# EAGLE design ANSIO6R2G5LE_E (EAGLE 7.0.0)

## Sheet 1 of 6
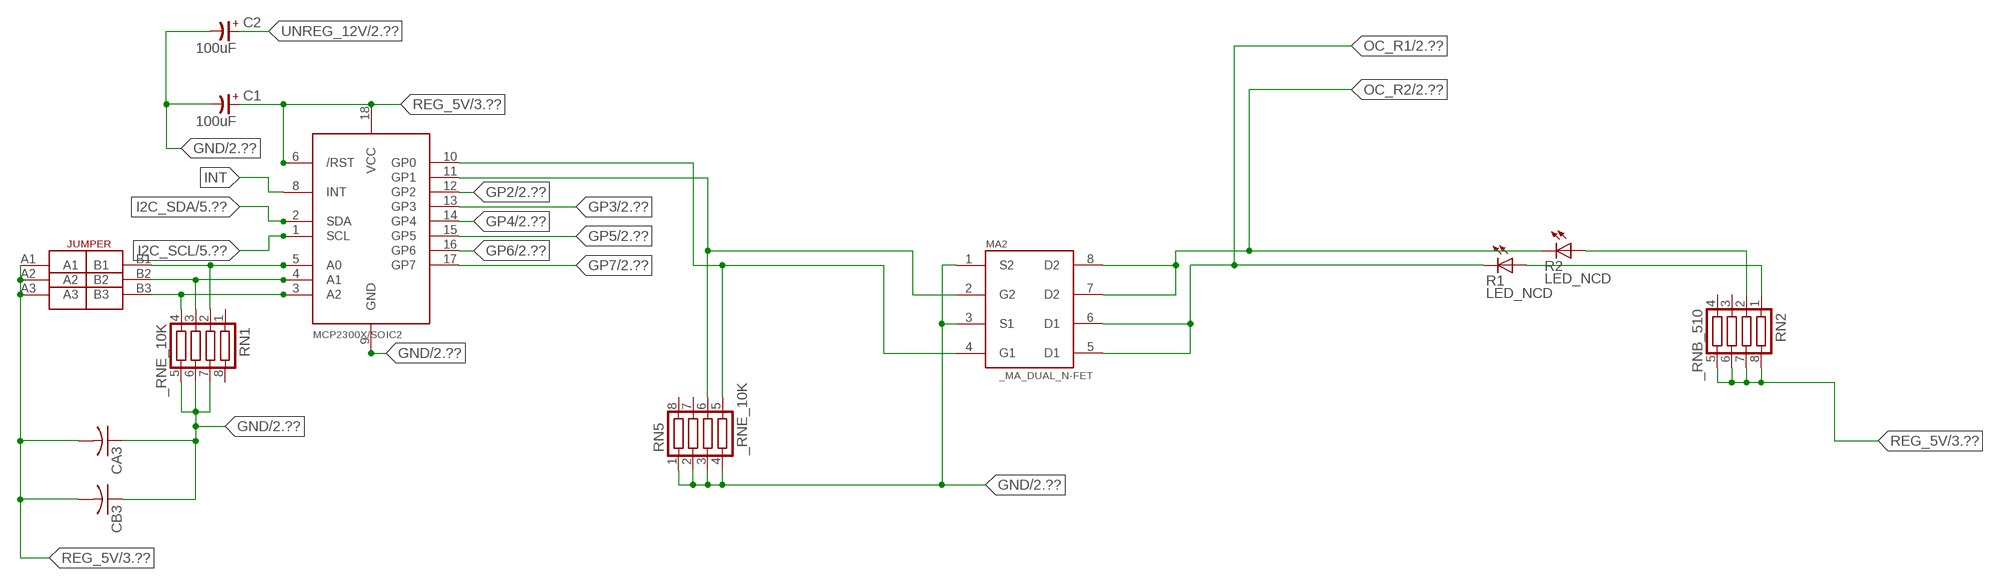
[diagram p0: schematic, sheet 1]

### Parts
C1  100uF  CP-E-025X060  [E-025X060]
C2  100uF  CP-E-025X060  [E-025X060]
CA3  CC1206KRX7R9BB104C1206K  [CC1206KRX7R9BB104]
CB3  TMK316F106ZL-TC1206K  [TMK316F106ZL-T]
IC2  MCP2300X/SO  [SO18W]
MA2  _MA_DUAL_N-FET  [_MA_DUAL_N-FET]
R1  LED_NCD  [CHIPLED_0603]
R2  LED_NCD  [CHIPLED_0603]
RN1  _RNE_10K  [RNE]
RN2  _RNB_510  [RNB]
RN5  _RNE_10K  [RNE]
U$18  JUMPER_3X2  [JUMPER_3X2]

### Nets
GND: C1.- C2.- CA3.1 CB3.1 IC2.9(GND) MA2.1(S2) MA2.3(S1) RN1.5 RN1.6 RN1.7 RN5.1 RN5.2 RN5.3 RN5.4 ; also sheet 2,3,4,5,6
GP2: IC2.12(GP2) ; also sheet 2
GP3: IC2.13(GP3) ; also sheet 2
GP4: IC2.14(GP4) ; also sheet 2
GP5: IC2.15(GP5) ; also sheet 2
GP6: IC2.16(GP6) ; also sheet 2
GP7: IC2.17(GP7) ; also sheet 2
I2C_SCL: IC2.1(SCL) ; also sheet 5,6
I2C_SDA: IC2.2(SDA) ; also sheet 5,6
INT: IC2.8(INT)
N$6: IC2.5(A0) RN1.2 U$18.B1
N$7: IC2.4(A1) RN1.3 U$18.B2
N$8: IC2.3(A2) RN1.4 U$18.B3
N$22: IC2.11(GP1) MA2.2(G2) RN5.6
N$23: IC2.10(GP0) MA2.4(G1) RN5.5
N$31: R2.A RN2.2
N$32: R1.A RN2.1
OC_R1: MA2.5(D1) MA2.6(D1) R1.C ; also sheet 2
OC_R2: MA2.7(D2) MA2.8(D2) R2.C ; also sheet 2
REG_5V: C1.+ CA3.2 CB3.2 IC2.6(/RST) IC2.18(VCC) RN2.5 RN2.6 RN2.7 RN2.8 U$18.A1 U$18.A2 U$18.A3 ; also sheet 3,4,5,6
UNREG_12V: C2.+ ; also sheet 2,3
Unconnected: RN1.1 RN1.8 RN2.3 RN2.4 RN5.7 RN5.8

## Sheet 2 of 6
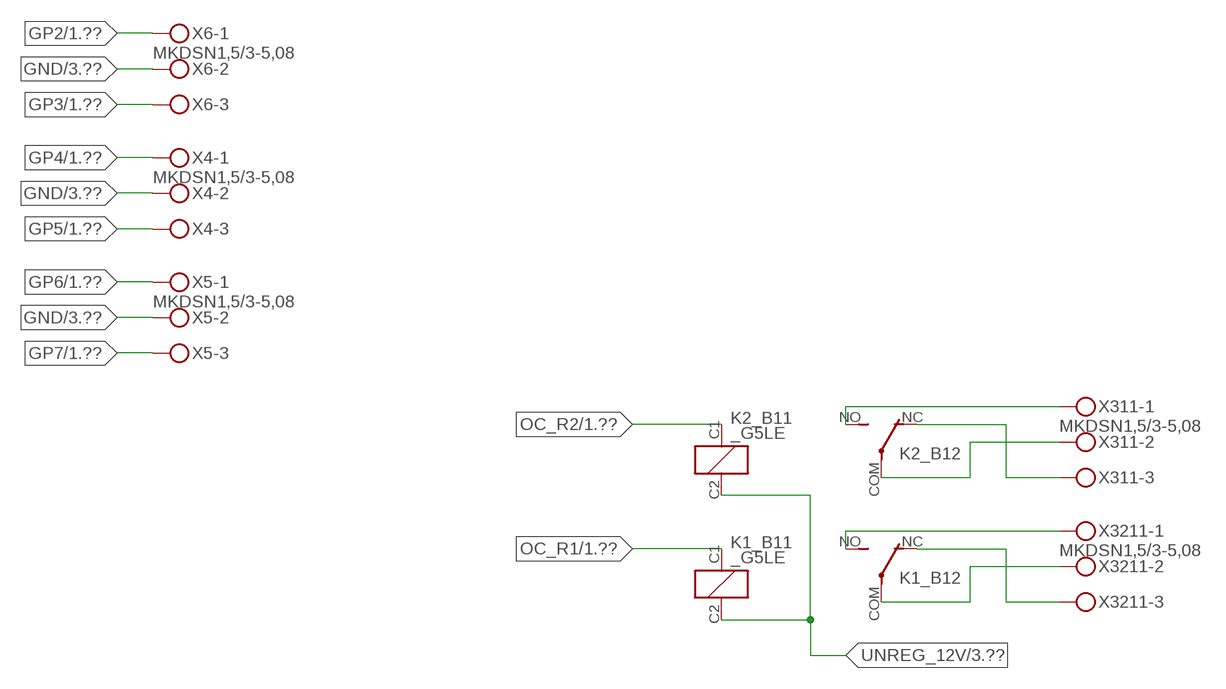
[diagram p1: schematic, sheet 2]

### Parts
K1_B1  _G5LE  [G5LE]
K2_B1  _G5LE  [G5LE]
X4  MKDSN1,5/3-5,08  [MKDSN1,5/3-5,08]
X5  MKDSN1,5/3-5,08  [MKDSN1,5/3-5,08]
X6  MKDSN1,5/3-5,08  [MKDSN1,5/3-5,08]
X311  MKDSN1,5/3-5,08  [MKDSN1,5/3-5,08]
X3211  MKDSN1,5/3-5,08  [MKDSN1,5/3-5,08]

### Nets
GND: X4.2 X5.2 X6.2 ; also sheet 1,3,4,5,6
GP2: X6.1 ; also sheet 1
GP3: X6.3 ; also sheet 1
GP4: X4.1 ; also sheet 1
GP5: X4.3 ; also sheet 1
GP6: X5.1 ; also sheet 1
GP7: X5.3 ; also sheet 1
N$221: K2_B1.NO(2:NO) X311.1
N$222: K2_B1.NC(2:NC) X311.3
N$223: K2_B1.COM(2:COM) X311.2
N$224: K1_B1.NO(2:NO) X3211.1
N$225: K1_B1.NC(2:NC) X3211.3
N$226: K1_B1.COM(2:COM) X3211.2
OC_R1: K1_B1.C1(1:C1) ; also sheet 1
OC_R2: K2_B1.C1(1:C1) ; also sheet 1
UNREG_12V: K1_B1.C2(1:C2) K2_B1.C2(1:C2) ; also sheet 1,3

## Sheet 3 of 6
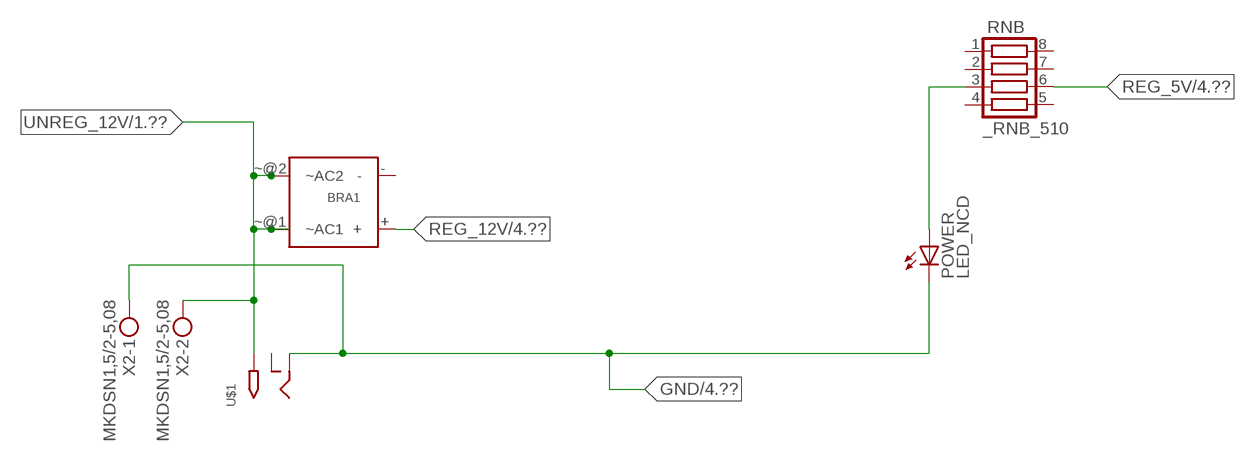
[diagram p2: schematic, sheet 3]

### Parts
BRA1  MB2S_  [MB2S]
POWER  LED_NCD  [CHIPLED_0603]
RNB  _RNB_510  [RNB]
U$1  2.1MMJACK  [PJ-102A]
X2  MKDSN1,5/2-5,08  [MKDSN1,5/2-5,08]

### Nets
GND: POWER.C U$1.RING X2.1 ; also sheet 1,2,4,5,6
N$1: POWER.A RNB.3
REG_5V: RNB.6 ; also sheet 1,4,5,6
REG_12V: BRA1.+ ; also sheet 4
UNREG_12V: BRA1.~@1(~AC1) BRA1.~@2(~AC2) U$1.TIP X2.2 ; also sheet 1,2
Unconnected: BRA1.- RNB.1 RNB.2 RNB.4 RNB.5 RNB.7 RNB.8 U$1.RING_SW

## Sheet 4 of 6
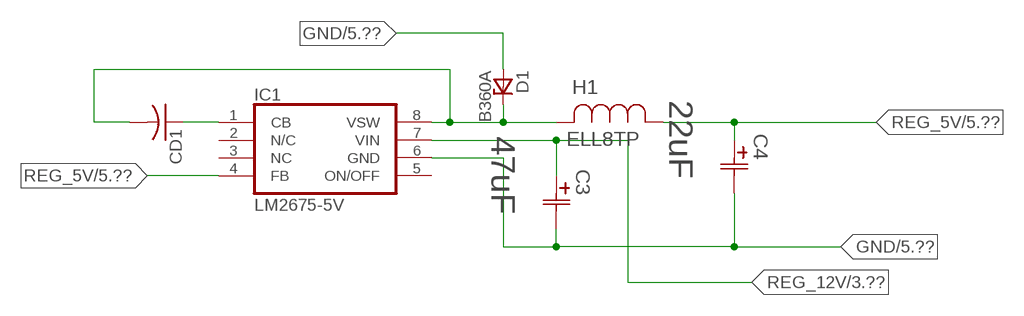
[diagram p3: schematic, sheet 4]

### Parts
C3  47uF  490-5463-6-NDCAP  [C2917(7343)-Y]
C4  22uF  490-5463-6-NDCAP  [C2917(7343)-Y]
CD1  _CD_10NF_50VC1206K  [_CD_10NF_50V]
D1  B360A  [DO214AC_ZENER]
H1  ELL8TP  [IND_ELL8TP]
IC1  LM2675-5V  LM2675  [SO-8]

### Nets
GND: C3.2(C2) C4.2(C2) D1.A IC1.6(GND) ; also sheet 1,2,3,5,6
N$9: CD1.2 D1.C H1.2 IC1.8(VSW)
N$10: CD1.1 IC1.1(CB)
REG_5V: C4.1(C1) H1.1 IC1.4(FB) ; also sheet 1,3,5,6
REG_12V: C3.1(C1) IC1.7(VIN) ; also sheet 3
Unconnected: IC1.2(N/C) IC1.5(ON/OFF)

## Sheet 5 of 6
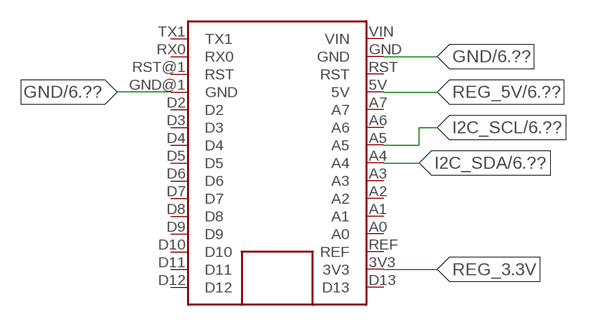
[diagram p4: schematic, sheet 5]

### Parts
FOR_NANO  ARDUINO_NANO  [ARDUINO_NANO]

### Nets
GND: FOR_NANO.GND FOR_NANO.GND@1(GND) ; also sheet 1,2,3,4,6
I2C_SCL: FOR_NANO.A5 ; also sheet 1,6
I2C_SDA: FOR_NANO.A4 ; also sheet 1,6
REG_3.3V: FOR_NANO.3V3
REG_5V: FOR_NANO.5V ; also sheet 1,3,4,6
Unconnected: FOR_NANO.A0 FOR_NANO.A1 FOR_NANO.A2 FOR_NANO.A3 FOR_NANO.A6 FOR_NANO.A7 FOR_NANO.D2 FOR_NANO.D3 FOR_NANO.D4 FOR_NANO.D5 FOR_NANO.D6 FOR_NANO.D7 FOR_NANO.D8 FOR_NANO.D9 FOR_NANO.D10 FOR_NANO.D11 FOR_NANO.D12 FOR_NANO.D13 FOR_NANO.REF FOR_NANO.RST FOR_NANO.RST@1(RST) FOR_NANO.RX0 FOR_NANO.TX1 FOR_NANO.VIN

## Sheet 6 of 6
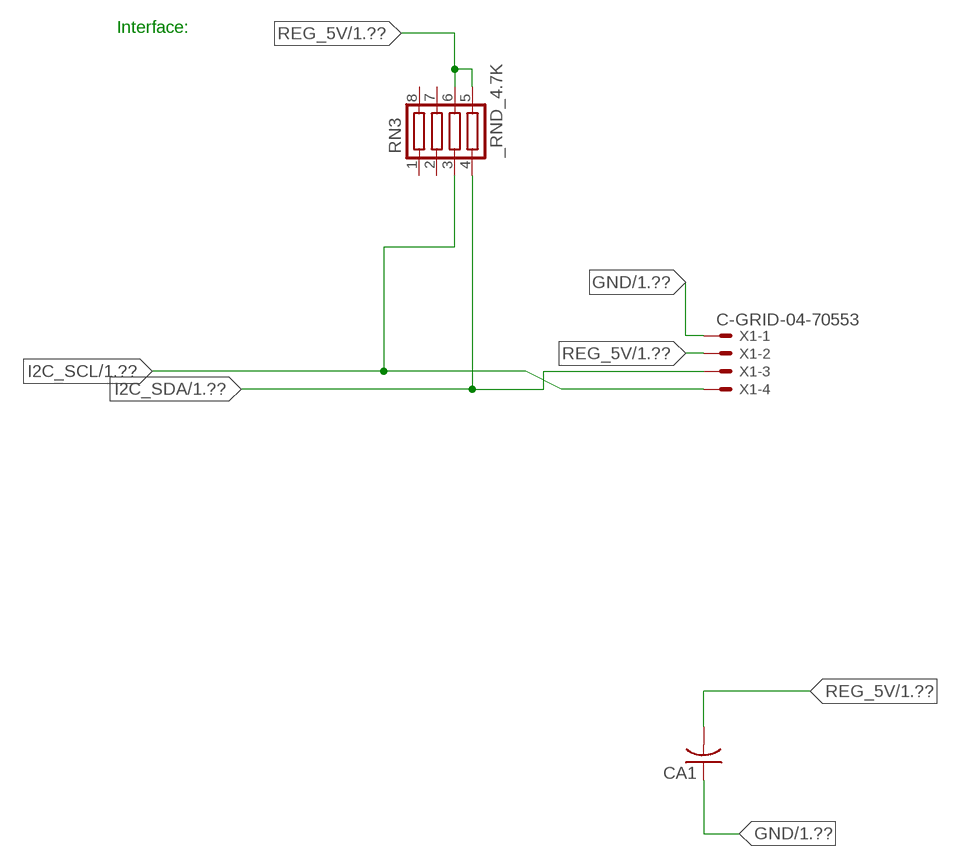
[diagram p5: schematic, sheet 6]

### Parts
CA1  CC1206KRX7R9BB104  [.1UF]
RN3  _RND_4.7K  [RND]
X1  C-GRID-04-70553  [70553-04]

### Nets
GND: CA1.1 X1.1 ; also sheet 1,2,3,4,5
I2C_SCL: RN3.3 X1.4 ; also sheet 1,5
I2C_SDA: RN3.4 X1.3 ; also sheet 1,5
REG_5V: CA1.2 RN3.5 RN3.6 X1.2 ; also sheet 1,3,4,5
Unconnected: RN3.1 RN3.2 RN3.7 RN3.8

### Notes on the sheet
- Interface:

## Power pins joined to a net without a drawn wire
NC: IC1.3(NC)

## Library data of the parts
BRA1 = NCD_ULTIMATE_LIBRARY:MB2S: Bridge Rectifier BRA MB2S 200V 500ma Digikey MB2S-TPMSTR-ND/MB2S-TP
C1 C2 = NCD_ULTIMATE_LIBRARY:CP-: Capacitors All Kinds POLARIZED CAP
C3 C4 = NCD_ULTIMATE_bhaskar:490-5463-6-ND: NCD CAP
CA1 CA3 = NCD_ULTIMATE_LIBRARY:CC1206KRX7R9BB104: Capacitor CA .1uF 50V SMT C1206K CC1206KRX7R9BB104
CB3 = NCD_ULTIMATE_LIBRARY:TMK316F106ZL-T: Capacitor CB 10uF SMT 1206 TMK316F106ZL-T
CD1 = NCD_ULTIMATE_LIBRARY:_CD_10NF_50V: Capacitor 10nF SMT
D1 = NCD_ULTIMATE_bhaskar:B360A: NCD DIODE B350A/B360A
FOR_NANO = NCD_ULTIMATE_CONNECTORS:ARDUINO_NANO
H1 = NCD_ULTIMATE_bhaskar:ELL8TP: NCD coil
IC1 = NCD_ULTIMATE_bhaskar:LM2675: LM2675 NCD http://www.ti.com/lit/ds/symlink/lm2675.pdf
IC2 = NCD_ULTIMATE_LIBRARY:MCP2300X: Semiconductor Port Expander I/O 8-Bit I2C MCP23008 Inexpensive i2c i/o expander - 8 general purpose i/o pins with optional pullups
K1_B1 K2_B1 = NCD_ULTIMATE_LIBRARY:_G5LE: Relay 5A/10A SPDT; OC_FARNELL: unknown; OC_NEWARK: unknown
MA2 = NCD_ULTIMATE_LIBRARY:_MA_DUAL_N-FET: FET Dual N-Channel 8-SOIC NMOSFET Digikey 785-1064-2-ND/AO4842
POWER = NCD_ULTIMATE_bhaskar:LED_NCD
R1 R2 = NCD_ULTIMATE_LIBRARY:LED_NCD: LED Digikey 754-1132-2-ND/APT2012SRCPRV
RN1 RN5 = NCD_ULTIMATE_LIBRARY:_RNE_10K: Resistor Array RNE SMT 10K x 4 Single Resistor Source: http://www.ctscorp.com/components/Datasheets/CTSChipArrayDs.pdf Digikey 742C083103JPTR-ND/742C083103JP; OC_FARNELL: unknown; OC_NEWARK: unknown
RN2 RNB = NCD_ULTIMATE_LIBRARY:_RNB_510: Resistor Array RNB SMT 510 x 4 Single Resistor Source: http://www.ctscorp.com/components/Datasheets/CTSChipArrayDs.pdf Digikey 742C083511JPTR-ND/ 742C083511JP; OC_FARNELL: unknown; OC_NEWARK: unknown
RN3 = NCD_ULTIMATE_LIBRARY:_RND_4.7K: Resistor Array RND SMT 4.7K x 4 Single Resistor Source: http://www.ctscorp.com/components/Datasheets/CTSChipArrayDs.pdf Digikey 742C083472JPTR-ND/742C083472JP; OC_FARNELL: unknown; OC_NEWARK: unknown
U$1 = NCD_ULTIMATE_CONNECTORS:2.1MMJACK: 2.1mm x 5.5mm DC jack with internal switch. Digikey part #PJ-102A, 4UCON part #05537 By microbuilder.eu
U$18 = NCD_ULTIMATE_CONNECTORS:JUMPER_3X2
X1 = NCD_ULTIMATE_CONNECTORS:C-GRID-04: CONNECTOR 4-Pos I2C wire to board 2.54 mm (0.100") pitch header Digikey WM1342-ND/0015912045; OC_FARNELL: unknown; OC_NEWARK: unknown
X2 = NCD_ULTIMATE_CONNECTORS:MKDSN1,5/2-5,08: MKDSN 1,5/ 2-5,08 Printklemme
X4-X6 X311 X3211 = NCD_ULTIMATE_CONNECTORS:MKDSN1,5/3-5,08: MKDSN 1,5/ 3-5,08 Printklemme Nennstrom: 13,5 A Nennspannung: 250 V Rastermaß: 5,08 mm Polzahl: 3 Anschlussart: Schraubanschluss Montage: Löten Anschlussrichtung Leiter/Platine: 0 ° Artikelnummer: 1729131 Source: http://eshop.phoenixcontact.com .. 1729131.pdf

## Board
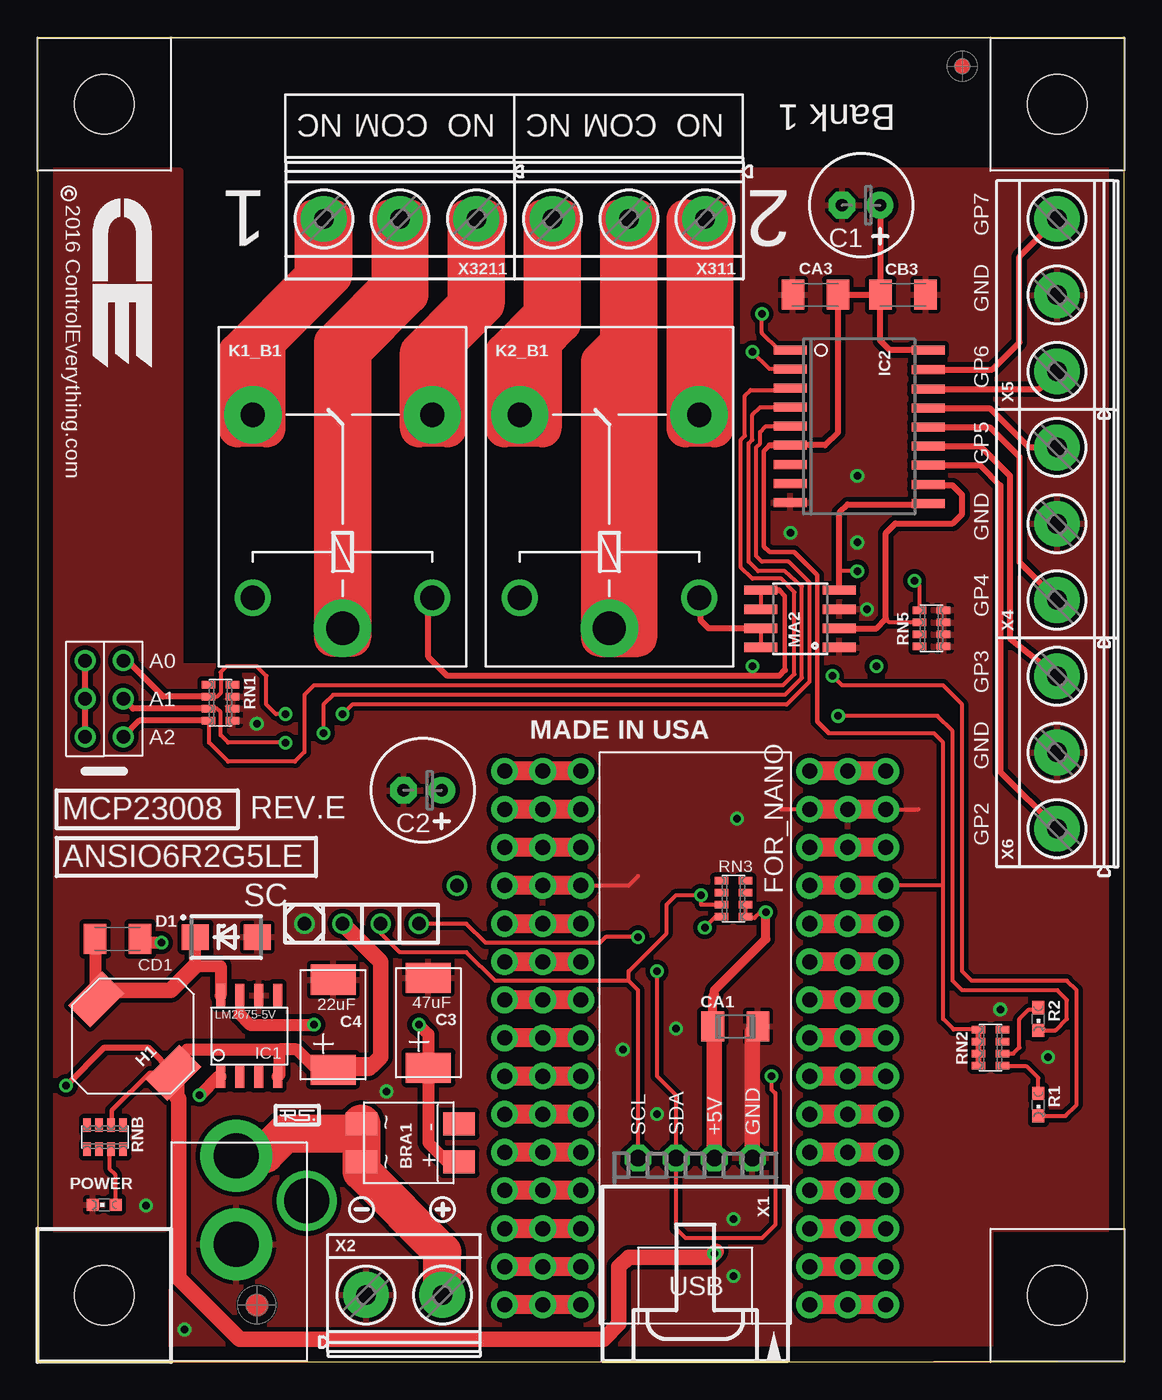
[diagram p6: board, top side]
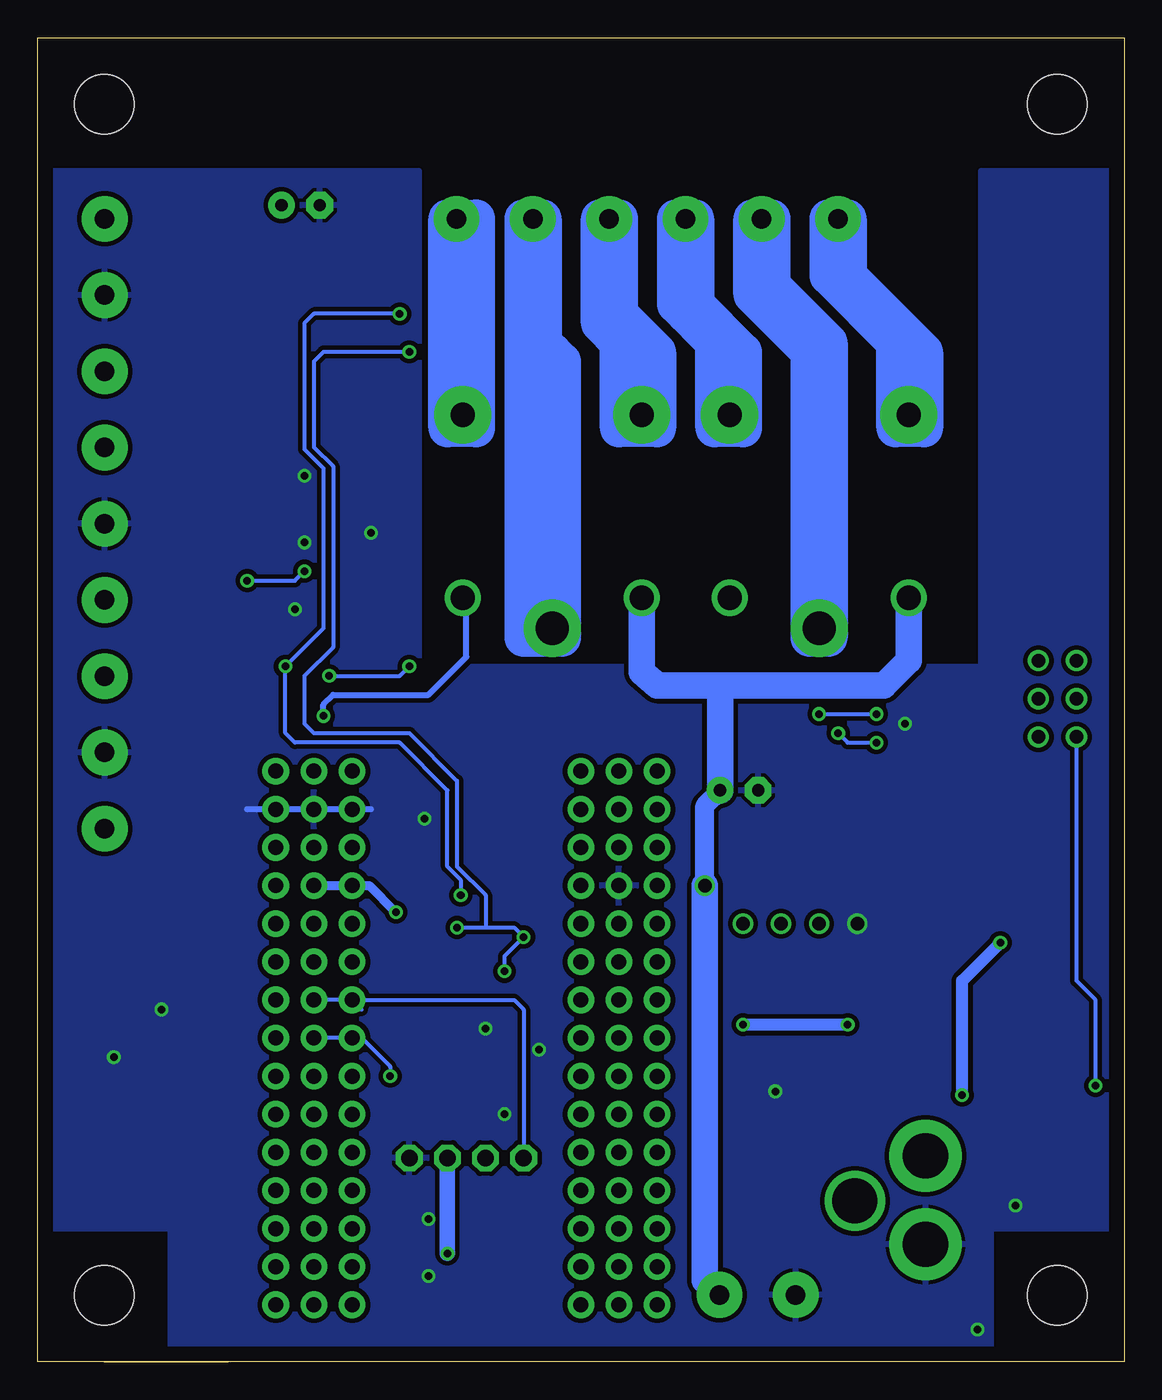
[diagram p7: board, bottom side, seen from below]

Size 72.39 x 88.27 mm. Coordinates in mm from the lower left corner, seen from the top.
Outline: 0,68.89 0,67.95
Outline: 0,67.95 0,0 59.69,0
Outline: 59.69,0 72.39,0 72.39,88.27 0,88.27 0,67.95
Outline: 67.94,0 59.69,0
Copper layers (1*16): Top 0.035mm / dielectric 1.5mm / Bottom 0.035mm
Design rules "default": minimum track width 10mil, minimum drill 24mil, track to track 8mil, track to pad 8mil, pad to pad 8mil, via to via 8mil, smd to smd 8mil, copper to edge 40mil, drill to drill 8mil, minimum pad ring 10mil, minimum via ring 8mil, stop-mask expansion 4mil, vias tented up to drill 0mil, thermal gap 10mil
Holes 3.96 mm at 4.45,4.44 4.45,4.44 4.45,4.44 4.45,4.44

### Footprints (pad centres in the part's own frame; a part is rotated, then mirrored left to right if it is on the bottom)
MB2S = smd 1.55 x 2.1: + 0,-6.5; - 2.54,-6.5; ~@1 0,0; ~@2 2.54,0
E-025X060 = drill 0.813 pad 1.778: + -1.27,0 | drill 0.813 pad 1.778 octagon: - 1.27,0
C2917(7343)-Y = smd 2 x 3: 1 -3,0; 2 3,0
.1UF = smd 1.5 x 2: 1 -1.5,0; 2 1.5,0
CC1206KRX7R9BB104 = smd 1.5 x 2: 1 -1.5,0; 2 1.5,0
TMK316F106ZL-T = smd 1.5 x 2: 1 -1.5,0; 2 1.5,0
_CD_10NF_50V = smd 1.5 x 2: 1 -1.5,0; 2 1.5,0
DO214AC_ZENER = smd 1.8 x 1.7: A 2.05,0; C -2.05,0
ARDUINO_NANO = drill 1 pad 1.778: 3V1 -2.54,-2.54; 3V3 0,-2.54; 5V 0,-27.94; 5V1 -2.54,-27.94; A0 0,-7.62; A1 0,-10.16; A2 0,-12.7; A3 0,-15.24; A4 0,-17.78; A5 0,-20.32; A6 0,-22.86; A7 0,-25.4; A8 -2.54,-7.62; A9 -2.54,-10.16; A10 -2.54,-12.7; A11 -2.54,-15.24; A12 -2.54,-17.78; A13 -2.54,-20.32; A14 -2.54,-22.86; A15 -2.54,-25.4; D1 -2.54,0; D2 20.32,-25.4; D3 20.32,-22.86; D4 20.32,-20.32; D5 20.32,-17.78; D6 20.32,-15.24; D7 20.32,-12.7; D8 20.32,-10.16; D9 20.32,-7.62; D10 20.32,-5.08; D11 20.32,-2.54; D12 20.32,0; D13 0,0; D14 22.86,0; D15 22.86,-2.54; D16 22.86,-5.08; D17 22.86,-7.62; D18 22.86,-10.16; D19 22.86,-12.7; D20 22.86,-15.24; D21 22.86,-17.78; D22 22.86,-20.32; D23 22.86,-22.86; D24 22.86,-25.4; GND 0,-33.02; GND1 -2.54,-33.02; GND@1 20.32,-27.94; GND@2 22.86,-27.94; P$16 2.54,0; P$17 2.54,-2.54; P$18 2.54,-5.08; P$19 2.54,-7.62; P$20 2.54,-10.16; P$21 2.54,-12.7; P$22 2.54,-15.24; P$23 2.54,-17.78; P$24 2.54,-20.32; P$25 2.54,-22.86; P$26 2.54,-25.4; P$27 2.54,-27.94; P$28 2.54,-30.48; P$29 2.54,-33.02; P$30 2.54,-35.56; P$31 17.78,0; P$32 17.78,-2.54; P$33 17.78,-5.08; P$34 17.78,-7.62; P$35 17.78,-10.16; P$36 17.78,-12.7; P$37 17.78,-15.24; P$38 17.78,-17.78; P$39 17.78,-20.32; P$40 17.78,-22.86; P$41 17.78,-25.4; P$42 17.78,-27.94; P$43 17.78,-30.48; P$44 17.78,-33.02; P$45 17.78,-35.56; REF 0,-5.08; REF1 -2.54,-5.08; RST 0,-30.48; RST1 -2.54,-30.48; RST@1 20.32,-30.48; RST@2 22.86,-30.48; RX0 20.32,-33.02; RX1 22.86,-33.02; TX1 20.32,-35.56; TX2 22.86,-35.56; VIN 0,-35.56; VIN1 -2.54,-35.56
IND_ELL8TP = smd 2.054 x 3.2 rotated 45: 1 -2.442,-2.696; 2 2.442,2.442
SO-8 = smd 0.6 x 1.55: 1 -1.905,-2.69; 2 -0.635,-2.69; 3 0.635,-2.69; 4 1.905,-2.69; 5 1.905,2.71; 6 0.635,2.71; 7 -0.635,2.71; 8 -1.905,2.71
SO18W = smd 0.6 x 2.2: 1 -4.445,-4.6; 2 -3.175,-4.6; 3 -1.905,-4.6; 4 -0.635,-4.6; 5 0.635,-4.6; 6 1.905,-4.6; 7 3.175,-4.6; 8 4.445,-4.6; 9 5.715,-4.6; 10 5.775,4.6; 11 4.505,4.6; 12 3.235,4.6; 13 1.965,4.6; 14 0.695,4.6; 15 -0.575,4.6; 16 -1.845,4.6; 17 -3.145,4.6; 18 -4.445,4.6
G5LE = drill 1.6: C1 -7.493,-5.969; C2 -7.493,5.969 | drill 2.2 pad 3.81: COM -9.525,0 | drill 1.6 pad 3.81: NC 4.699,5.969; NO 4.699,-5.969
_MA_DUAL_N-FET = smd 0.61 x 2.21: 1 -1.905,-2.616; 2 -0.635,-2.616; 3 0.635,-2.616; 4 1.905,-2.616; 5 1.905,2.616; 6 0.635,2.616; 7 -0.635,2.616; 8 -1.905,2.616
CHIPLED_0603 = smd 0.8 x 0.8: A 0,-0.75; C 0,0.75
CHIPLED_0603' = smd 0.8 x 0.876: A 0,-0.75; C 0,0.75
RNE = smd 0.5 x 0.9: 1 -1.2,-0.8; 2 -0.4,-0.8; 3 0.4,-0.8; 4 1.2,-0.8; 5 1.2,0.8; 6 0.4,0.8; 7 -0.4,0.8; 8 -1.2,0.8
RNB = smd 0.5 x 0.9: 1 -1.2,-0.8; 2 -0.4,-0.8; 3 0.4,-0.8; 4 1.2,-0.8; 5 1.2,0.8; 6 0.4,0.8; 7 -0.4,0.8; 8 -1.2,0.8
RND = smd 0.5 x 0.9: 1 -1.2,-0.8; 2 -0.4,-0.8; 3 0.4,-0.8; 4 1.2,-0.8; 5 1.2,0.8; 6 0.4,0.8; 7 -0.4,0.8; 8 -1.2,0.8
PJ-102A = drill 3 pad 4.8: RING 0.1,-3.39; TIP 0.1,-9.29 | drill 3 pad 3.251: RING_SW -4.6,-6.29
PCB_MOUNTING_HOLE = hole 3.962: 4.445,4.445
JUMPER_3X2 = drill 0.9: A1 0,5.08; A2 0,2.54; A3 0,0; B1 2.54,5.08; B2 2.54,2.54; B3 2.54,0
70553-04 = drill 1.1 pad 1.778 octagon: 1 -3.81,-7.62; 2 -1.27,-7.62; 3 1.27,-7.62; 4 3.81,-7.62
MKDSN1,5/2-5,08 = drill 1.3 pad 3.048: 1 -2.561,0.025; 2 2.519,0.025
MKDSN1,5/3-5,08 = drill 1.3 pad 3.048: 1 -7.641,0.025; 2 -2.561,0.025; 3 2.519,0.025

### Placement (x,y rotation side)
BRA1  21.59,13.33 90 top
C1  54.86,77.09 180 top
C2  25.65,38.1 180 top
C3  26.04,22.61 90 top
C4  19.68,22.48 90 top
CA1  46.48,22.35 180 top
CA3  51.82,71.12 0 top
CB3  57.66,71.12 180 top
CD1  5.33,28.19 180 top
D1  12.57,28.32 0 top
FOR_NANO  53.98,3.81 180 top
H1  6.35,21.72 90 top
IC1  14.1,21.72 0 top
IC2  54.74,62.99 270 top
K1_B1  20.32,58.42 90 top
K2_B1  38.1,58.42 90 top
MA2  50.8,49.53 90 top
POWER  4.45,10.48 90 top
R1  LED_NCD  [CHIPLED_0603']  66.67,17.14 180 top
R2  LED_NCD  [CHIPLED_0603']  66.67,22.86 180 top
RN1  12.19,43.94 270 top
RN2  63.5,20.95 90 top
RN3  46.35,30.86 270 top
RN5  59.56,48.89 90 top
RNB  4.51,14.99 0 top
U$1  13.34,4.44 180 top
U$2  [VISION_REF15]  14.61,3.81 0 top
U$3  [ICON_MINUS]  21.59,10.16 180 top
U$4  PCB_MOUNTING_HOLE  [PCB_MOUNTING_HOLE]  72.39,79.38 90 top
U$5  [ICON_PLUS]  26.99,10.16 90 top
U$6  PCB_MOUNTING_HOLE  [PCB_MOUNTING_HOLE]  72.39,0 90 top
U$11  PCB_MOUNTING_HOLE  [PCB_MOUNTING_HOLE]  8.89,79.38 90 top
U$18  3.17,41.66 0 top
U$19  [VISION_REF10]  61.59,86.36 0 top
U$21  [ICON_USA]  32.77,41.53 0 top
X1  43.81,5.97 180 top
X2  24.45,4.44 0 top
X4  67.94,58.42 90 top
X5  67.94,73.66 90 top
X6  67.94,43.18 90 top
X311  36.83,76.2 180 top
X3211  21.59,76.2 180 top

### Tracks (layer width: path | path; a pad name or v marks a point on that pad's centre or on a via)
GND  (via drill 0.5, 0.9)
  Top 0.254: 36.2,31.75 39.37,31.75 40.01,32.38 | FOR_NANO.GND@1 32.38,31.75 | 49.53,36.83 56.52,36.83 58.67,36.83
  Top 1.016: X1.1 47.62,21.99
  Bottom 0.254: 51.44,36.83 FOR_NANO.GND
  Bottom 0.305: 50.42,36.83 51.44,36.83
  Bottom 0.406: 50.16,36.83 50.42,36.83 58.42,36.83
  other vias: 54.61,54.61 54.61,59.05 64.14,23.49 67.31,20.32 50.16,55.24 55.24,50.16 14.61,42.55 9.78,2.16 17.78,29.21 41.27,16.51 46.35,9.52 46.61,36.2 46.35,5.71 42.55,22.23 38.99,20.83 7.24,10.41 23.24,18.03
  pour Bottom (isolate 0.305): -1.27,8.89 8.89,8.89 8.89,0 63.5,0 63.5,8.89 71.75,8.89 71.75,79.38 46.99,79.38 46.99,46.35 9.53,46.35 9.53,79.38 -1.27,79.38
  pour Top (isolate 0.305): -2.54,8.89 8.89,8.89 8.89,0 63.5,0 63.5,8.89 71.75,8.89 71.75,79.38 46.99,79.38 46.99,46.35 9.53,46.35 9.53,79.38 -2.54,79.38
GP2
  Top 0.406: IC2.12 62.8,59.76 64.14,58.42 64.14,39.32 X6.1
GP3
  Top 0.406: IC2.13 62.8,61.03 64.77,59.05 64.77,48.21 X6.3
GP4
  Top 0.406: IC2.14 63.43,62.3 65.41,60.32 65.41,53.29 X4.1
GP5
  Top 0.406: IC2.15 63.43,63.57 66.04,60.96 67.9,60.96 X4.3
GP6
  Top 0.406: IC2.16 66.74,64.84 X5.1
GP7
  Top 0.406: IC2.17 63.6,66.14 65.41,67.95 65.41,73.66 X5.3
I2C_SCL  (via drill 0.5, 0.9)
  Top 0.254: IC2.1 49.4,67.44 48.26,68.58 v48.26,69.85 | 39.37,25.4 40.01,24.77 X1.4 | 39.37,25.4 30.48,25.4 28.57,27.3 24.13,27.3 22.86,28.58 v22.86,29.21 | RN3.3 45.54,30.48 44.2,30.48 v44.2,31.12 42.55,31.12 41.91,30.48 41.91,28.58 39.37,26.04 39.37,25.4
  Bottom 0.254: v48.26,69.85 53.98,69.85 54.61,69.22 54.61,60.83 53.34,59.56 53.34,48.89 v55.88,46.35 55.88,41.91 55.24,41.27 48.26,41.27 45.09,38.1 45.09,33.02 44.2,32.13 v44.2,31.12 | 50.8,23.49 51.44,24.13 | 51.44,24.13 FOR_NANO.A5 | 51.44,24.13 40.64,24.13 40.01,23.49 X1.4
I2C_SDA  (via drill 0.5, 0.9)
  Top 0.254: IC2.2 48.77,66.17 v47.62,67.31 | RN3.4 45.16,29.66 v44.45,28.96 | 40,28.33 v40.01,28.32 37.85,28.32 37.47,27.94 29.84,27.94 28.57,29.21 v25.4,29.21 | v41.27,26.04 41.27,19.05 42.55,17.78 X1.3 42.55,8.89 43.18,8.25 48.26,8.25 49.15,9.14 49.15,17.91 48.9,18.16 v48.9,19.05
  Bottom 0.254: v47.62,67.31 53.34,67.31 53.98,66.67 53.98,60.96 52.7,59.69 52.7,47.62 54.61,45.72 54.61,42.55 53.98,41.91 47.62,41.91 44.45,38.73 44.45,33.02 42.55,31.12 42.55,28.96 | v44.45,28.96 42.55,28.96 | 42.55,28.96 40.64,28.96 v40.01,28.32 41.27,27.05 v41.27,26.04 | v48.9,19.05 48.9,19.68 50.8,21.59 FOR_NANO.A4
N$1
  Top 0.254: POWER.A 5.2,12.46 4.83,12.83 4.83,14.1 RNB.3
  Top 0.406: 4.95,14.14 RNB.3
N$6  (via drill 0.5)
  Top 0.254: v20.32,43.18 20.95,43.81 49.91,43.81 51.44,45.34 51.44,51.94 50.04,53.34 48.26,53.34 47.88,53.72 47.88,60.96 48.13,61.21 48.13,61.98 48.51,62.36 IC2.5 50.01,62.23 | v16.51,43.18 15.88,43.18 15.24,43.81 15.24,45.72 14.61,46.35 12.57,46.35 12.19,45.97 12.19,44.58 11.94,44.32 11.41,44.32 RN1.2
  Top 0.406: RN1.2 8.36,44.34 5.97,46.74 U$18.B1
  Bottom 0.254: v20.32,43.18 v16.51,43.18
N$7  (via drill 0.5)
  Top 0.254: v19.05,41.91 19.05,43.81 19.68,44.45 49.78,44.45 50.93,45.59 50.93,51.69 49.78,52.7 48.01,52.7 47.37,53.34 47.37,61.21 47.62,61.47 47.62,63.12 48.13,63.63 IC2.4 50.01,63.5 | v16.51,41.27 12.7,41.27 12.19,41.78 12.19,43.31 11.94,43.56 11.41,43.56 RN1.3
  Top 0.406: RN1.3 6.37,43.54 U$18.B2
  Bottom 0.254: v19.05,41.91 18.41,41.27 v16.51,41.27
N$8
  Top 0.254: RN1.4 11.43,42.7 11.43,41.27 12.7,40.01 17.14,40.01 17.78,40.64 17.78,44.45 18.41,45.09 49.66,45.09 50.42,45.85 50.42,51.31 49.53,52.2 47.62,52.2 46.86,52.96 46.86,61.47 47.12,61.72 47.12,64.39 47.5,64.77 50.01,64.77 IC2.3
  Top 0.406: RN1.4 6.79,42.74 U$18.B3
N$9
  Top 0.813: H1.2 3.88,24.77 | D1.C 10.52,26.4 12.19,26.38 IC1.8 | CD1.2 3.83,24.15 4.45,24.77
  Top 1.016: 3.88,24.77 4.45,24.77 8.89,24.77 10.52,26.4
N$10  (via drill 0.5)
  Top 0.813: IC1.1 12.04,19.03 v10.79,17.78 | v8.26,27.94 7.72,27.94 CD1.1
  Bottom 0.813: v10.79,17.78 10.79,25.4 v8.26,27.94
N$22
  Top 0.254: RN5.6 56.75,49.29 56.52,49.53
  Top 0.406: MA2.2 55.88,48.89 56.52,49.53 56.52,55.24 57.15,55.88 60.96,55.88 61.59,56.52 61.59,57.78 60.96,58.42 59.4,58.42 IC2.11
N$23  (via drill 0.5)
  Top 0.254: RN5.5 58.76,51.73 v58.42,52.07 | v54.61,52.7 53.42,52.7
  Top 0.406: MA2.4 53.42,52.7 53.42,56.59 53.98,57.15 59.27,57.15 IC2.10
  Bottom 0.254: v58.42,52.07 55.24,52.07 v54.61,52.7
N$31
  Top 0.254: RN2.2 65,20.55 65.41,20.95 65.41,22.86 66.04,23.49 66.56,23.49 R2.A
N$32
  Top 0.254: R1.A 66.67,18.92 65.91,19.68 64.37,19.68 RN2.1
N$221
  Top 2.54: X311.1 44.47,63.52 K2_B1.NO
N$222
  Top 2.54: X311.3 34.31,69.24 32.38,67.31 32.38,63.37 K2_B1.NC
N$223
  Top 2.54: X311.2 39.39,50.19 K2_B1.COM
N$224
  Top 2.54: X3211.1 29.23,70.51 26.04,67.31 26.04,63.37 K1_B1.NO
N$225
  Top 2.54: X3211.3 19.07,72.41 13.97,67.31 13.97,63.5 K1_B1.NC
N$226
  Top 2.54: X3211.2 24.15,71.78 20.32,67.95 K1_B1.COM
N$322
  Top 2.54: 44.47,76.17 44.47,63.52 44.07,63.12
N$323
  Top 2.54: 34.31,76.17 34.31,69.24 32.38,67.31 32.38,63.37 32.13,63.12
N$324
  Top 2.54: 39.39,76.17 39.39,50.19 38.1,48.89
N$325
  Top 2.54: 29.23,76.17 29.23,70.51 26.67,67.95 26.67,63.5 26.29,63.12
N$326
  Top 2.54: 19.07,76.17 19.07,72.41 14.61,67.95 14.61,63.37 14.35,63.12
N$327
  Top 2.54: 24.15,76.17 24.15,71.78 20.32,67.95 20.32,48.89
N$328
  Bottom 2.54: 20.32,48.89 20.32,67.31 24.13,71.12 24.13,76.15 24.15,76.17
N$329
  Bottom 2.54: 14.35,63.12 14.35,67.69 19.05,72.39 19.05,76.15 19.07,76.17
N$330
  Bottom 2.54: 26.29,63.12 26.29,66.93 29.21,69.85 29.21,76.15 29.23,76.17
N$331
  Bottom 2.54: 44.07,63.12 44.07,65.66 44.45,66.04 44.45,76.15 44.47,76.17
N$333
  Bottom 2.54: 32.13,63.12 32.13,66.42 34.29,68.58 34.29,76.15 34.31,76.17
N$334
  Bottom 2.54: 38.1,48.89 38.1,67.31 39.37,68.58 39.37,76.15 39.39,76.17
N$342
  Top 2.54: 45.09,76.2 45.09,62.23 43.18,62.23 43.18,76.2 45.09,76.2
N$343
  Top 2.54: 40.01,76.2 40.01,48.26 37.47,48.26 37.47,66.67 38.73,67.95 38.73,76.2 40.01,76.2
N$344
  Top 2.54: 34.92,76.2 34.92,69.22 33.66,67.95 33.66,62.23 31.11,62.23 31.11,67.31 33.66,69.85 33.66,76.2 34.92,76.2
N$345
  Top 2.54: 29.21,76.2 29.84,76.2 29.84,70.48 27.3,67.95 27.3,62.23 25.4,62.23 25.4,67.31 28.57,70.48 | 29.21,71.12 29.21,76.2 | 29.21,76.2 28.57,76.2 28.57,69.85
N$346
  Top 2.54: 24.77,71.75 24.77,76.2 24.13,76.2 | 24.77,71.75 23.5,70.48 | 23.5,70.48 20.95,67.95 20.95,67.31 | 20.95,67.31 20.95,48.26 19.68,48.26 19.68,67.95 24.13,72.39 24.13,76.2 | 24.13,76.2 23.5,76.2 23.5,70.48 | 24.77,71.75 24.77,71.12 20.95,67.31
N$347
  Top 2.54: 19.68,76.2 19.68,72.39 15.24,67.95 15.24,62.23 13.34,62.23 13.34,67.31 18.41,72.39 18.41,76.2 19.68,76.2
N$348
  Bottom 2.54: 19.05,76.2 18.41,76.2 18.41,72.39 13.34,67.31 13.34,62.23 15.24,62.23 15.24,67.95 19.68,72.39 19.68,76.2
N$349
  Bottom 2.54: 23.5,76.2 23.5,71.75 19.68,67.95 19.68,48.26 20.95,48.26 20.95,67.31 24.77,71.12 24.77,76.2 23.5,76.2
N$350
  Bottom 2.54: 28.57,76.2 28.57,70.48 25.4,67.31 25.4,62.23 27.3,62.23 27.3,67.95 29.84,70.48 29.84,76.2 28.57,76.2
N$351
  Bottom 2.54: 33.66,76.2 33.66,69.85 31.11,67.31 31.11,62.23 33.66,62.23 33.66,67.95 34.92,69.22 34.92,76.2 33.66,76.2
N$352
  Bottom 2.54: 38.73,76.2 38.73,67.95 37.47,66.67 37.47,48.26 40.01,48.26 40.01,76.2 38.73,76.2
N$353
  Bottom 2.54: 45.09,76.2 43.18,76.2 43.18,62.23 45.09,62.23 45.09,76.2
OC_R1  (via drill 0.5)
  Top 0.254: MA2.5 MA2.6 | R1.C 68.47,16.39 69.22,17.14 69.22,24.77 68.58,25.4 62.23,25.4 61.59,26.04 61.59,43.81 60.33,45.09 53.59,45.09 v52.96,45.72 | v47.62,46.35 47.62,45.72
  Top 0.305: 49.4,51.43 49.78,51.05 49.78,46.1
  Top 0.406: MA2.5 49.4,51.43 | 49.78,46.1 49.4,45.72 47.62,45.72 27.3,45.72 26.04,46.99 26.04,50.67 K1_B1.C1
  Bottom 0.254: v52.96,45.72 48.26,45.72 v47.62,46.35
OC_R2  (via drill 0.5)
  Top 0.254: MA2.7 MA2.8 | R2.C 67.83,22.11 68.58,22.86 68.58,24.13 67.94,24.77 61.59,24.77 60.96,25.4 60.96,42.04 59.94,43.05 v53.34,43.05
  Top 0.406: MA2.7 44.7,48.89 44.2,49.4 44.2,50.8 K2_B1.C1
  Bottom 0.406: v53.34,43.05 53.34,43.81 52.7,44.45 46.35,44.45 43.81,46.99 43.81,50.67 K2_B1.C1
REG_5V  (via drill 0.5, 0.9)
  Top 0.254: RN2.5 61.03,22.16 60.33,22.86 60.33,31.75 | 60.33,31.75 60.33,41.27 59.69,41.91 52.7,41.91 | RN3.6 RN3.5 47.23,29.59 47.75,29.59 48.13,29.97 v48.51,29.97 | 44.98,24.41 45.09,24.51 | 60.33,31.75 FOR_NANO.5V
  Top 0.305: 48.77,61.09 48.39,60.71 48.39,54.36 48.77,53.97 50.42,53.97 51.94,52.45 51.94,42.67 52.7,41.91 | H1.1 7.46,19.27 4.95,16.76 4.95,15.83 RNB.6
  Top 0.406: U$18.A3 U$18.A2 U$18.A1 | RN2.8 RN2.7 RN2.6 RN2.5 | 48.77,61.09 IC2.6 52.45,61.09 53.32,61.95 CA3.2 CB3.2 56.13,71.1 | IC2.18 56.77,67.44 56.13,68.07 56.13,71.1 | C1.+ 56.13,71.1 | v1.91,18.41 4.45,20.95 7.37,20.95 H1.1
  Top 0.61: CA1.2 44.98,24.41 | 45.09,24.51 45.09,24.77 48.51,28.19 v48.51,29.97
  Top 0.813: 16.13,20.83 9.96,20.83 H1.1 | 16.13,20.83 17.27,20.83 18.41,19.68 20.75,19.68 C4.1 | IC1.4 16.13,19.15 16.13,20.83
  Top 1.016: H1.1 9.27,18.41 9.27,17.65 9.4,17.53 9.4,5.59 13.46,1.52 37.72,1.52 38.73,2.54 38.73,6.35 39.37,6.98 44.83,6.98 v45.09,7.24 45.21,7.37 | 22.05,19.68 22.23,19.68 22.86,20.32 22.86,26.67 v20.32,29.21 | X1.2 45.09,22.25 CA1.2
  Top 1.27: 20.75,19.68 22.05,19.68
  Bottom 0.254: v1.91,18.41 1.91,24.13 3.17,25.4 U$18.A3
  Bottom 0.61: FOR_NANO.5V 50.29,31.75 v48.51,29.97
  Bottom 1.016: v45.09,7.24 X1.2
REG_12V  (via drill 0.5)
  Top 0.61: IC1.7 13.46,23.16 | 14.1,22.48 14.15,22.48
  Top 0.813: v18.41,22.48 14.15,22.48 13.46,23.16 | v25.4,22.48 26.04,21.84 C3.1 26.04,14.61 27.3,13.33 BRA1.+
  Bottom 0.813: v18.41,22.48 v25.4,22.48
UNREG_12V  (via drill 0.9)
  Top 2.54: X2.2 26.97,7.32 21.59,12.7 BRA1.~@1 21.59,15.24 | 21.59,15.24 BRA1.~@2 | U$1.TIP 15.14,13.87 16.51,15.24 21.59,15.24
  Bottom 1.27: v27.94,31.75 27.94,37.08 C2.+
  Bottom 1.778: 27.3,45.09 31.11,45.09 32.13,45.97 K2_B1.C2 | 27.3,45.09 16,45.09 14.35,46.74 K1_B1.C2 | C2.+ 26.92,44.7 27.3,45.09 | v27.94,31.75 27.94,5.44 X2.2

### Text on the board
tNames: Bank 1 | NC | COM | NO | NC | COM | NO | 1 | 2 | 2016 ControlEverything.com | GP7 | GND | GP6 | GP5 | GND | GP4 | A0 | GP3 | A1 | A2 | GND | MCP23008 | REV.E | GP2 | ANSIO6R2G5LE | SC | SCL | SDA | +5V | GND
